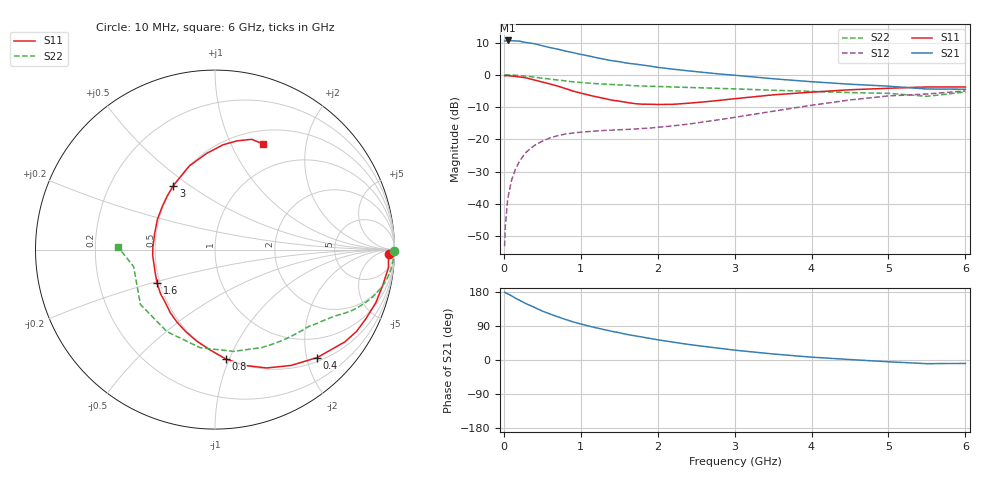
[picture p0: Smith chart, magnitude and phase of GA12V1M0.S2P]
! Infineon Technologies  Discrete & RF Semiconductors
! BF775
! Si NPN RF Bipolar Junction Transistor in SOT23
! VCE = 12 V  IC = 1 mA
! Common Emitter S-Parameters:  May  1996
# GHz  S  MA  R  50
!  f  S11  S21  S12  S22
! GHz  MAG  ANG  MAG  ANG  MAG  ANG  MAG  ANG
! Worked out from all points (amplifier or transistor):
!   36 points, 10 MHz to 6 GHz, reference 50 ohm
!   highest |S21| = 10.6 dB at 50 MHz (marker M1)
!   |S21| within 3 dB of that: start of sweep to 751.8 MHz
!   unconditionally stable (mu >= 1): 1.502 GHz to 3.35 GHz; 5.496499 GHz to 5.50935 GHz
!   at 250 MHz: K = 0.20, MSG = 17.7 dB, |S12| = -25.2 dB
!   at 1.4 GHz: K = 0.96, MSG = 10.8 dB, |S12| = -17.2 dB
!   at 6 GHz: K = 0.97, MSG = 0.3 dB, |S12| = -5.0 dB
!   S11 on the Smith chart (normalised r, x): 10 MHz: 43, -32; 400 MHz: 0.57, -2.20; 800 MHz: 0.50, -0.97; 1.6 GHz: 0.48, -0.21; 3 GHz: 0.50, +0.43; 6 GHz: 0.65, +1.33
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0.01  0.9707 -1.3  3.346 179.1  0.0022 90.8  0.9999 -0.4
0.02  0.9676 -2.5  3.326 177.6  0.0045 83.7  0.9958 -0.9
0.05  0.9717 -6.0  3.406 174.6  0.0118 86.2  0.9968 -2.3
0.1  0.9553 -12.1  3.37 169.5  0.0231 83.0  0.9916 -4.6
0.15  0.9439 -18.2  3.347 163.1  0.0342 78.0  0.9842 -6.9
0.2  0.9259 -24.2  3.328 158.1  0.045 74.9  0.9749 -9.1
0.3  0.8876 -35.4  3.15 147.6  0.0646 68.5  0.9491 -13.1
0.4  0.828 -46.6  3.031 138.6  0.0804 62.2  0.9177 -16.7
0.5  0.7721 -56.7  2.822 129.1  0.0934 57.2  0.8843 -19.8
0.6  0.7197 -66.4  2.64 121.4  0.1051 52.5  0.8573 -22.1
0.8  0.6122 -84.4  2.336 107.1  0.1206 45.9  0.8034 -26.2
0.9  0.5589 -92.9  2.203 100.6  0.1251 43.7  0.7783 -27.9
1.1  0.4857 -109.5  1.96 89.9  0.1316 40.5  0.7428 -31.0
1.3  0.4306 -125.4  1.749 80.4  0.1369 38.9  0.7176 -33.7
1.6  0.3719 -150.4  1.517 67.5  0.1421 39.0  0.688 -37.8
2.2  0.3481 164.8  1.222 47.1  0.1614 45.0  0.6472 -47.2
3  0.4255 123.0  0.984 26.0  0.2188 50.9  0.6046 -64.6
3.5  0.4884 106.9  0.868 15.9  0.2722 50.2  0.5765 -79.6
4.5  0.5857 85.6  0.714 1.2  0.407 40.1  0.5297 -120.4
5  0.6178 78.6  0.666 -4.7  0.4702 31.8  0.5158 -143.7
5.5  0.6475 71.6  0.602 -9.7  0.5032 21.8  0.4631 -168.2
6  0.6468 65.8  0.597 -9.0  0.5619 16.6  0.541 178.4
